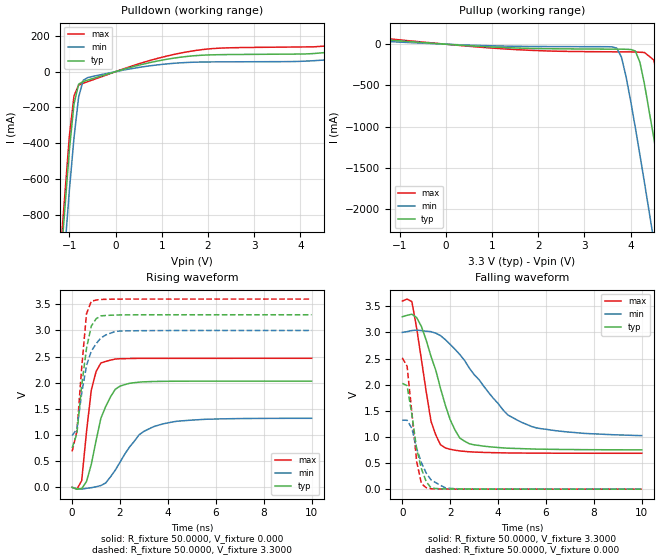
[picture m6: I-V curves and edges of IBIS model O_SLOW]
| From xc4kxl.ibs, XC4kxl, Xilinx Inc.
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|   Model O_SLOW
[Model]   O_SLOW
Model_type   Output
Polarity   Non-Inverting
Vmeas =   1.6500V
Cref =  50.0000pF
Rref =   1.0000M
Vref =  0.000V
C_comp   7.0000pF   6.0000pF   8.0000pF
[Temperature Range]   27.0000   100.0000   0.000
[Voltage Range]   3.3000V   3.0000V   3.6000V
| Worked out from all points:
|   slope of the pulldown table from 0 to 0.495 V, typ, clamps not added: 13.9 ohm
|   slope of the pullup table from 0 to 0.495 V, typ, clamps not added: 27.1 ohm
|   rising waveform, R_fixture 50.0000, V_fixture 0.000: 20-80 % time 708ps typ, 1.25ns min, 387ps max; typ from 0 V to 2.03 V
|   rising waveform, R_fixture 50.0000, V_fixture 3.3000: 20-80 % time 413ps typ, 515ps min, 309ps max; typ from 0.751 V to 3.3 V
|   falling waveform, R_fixture 50.0000, V_fixture 3.3000: 20-80 % time 1.03ns typ, 2.06ns min, 600ps max; typ from 3.3 V to 0.752 V
|   falling waveform, R_fixture 50.0000, V_fixture 0.000: 20-80 % time 461ps typ, 610ps min, 335ps max; typ from 2.02 V to 0 V
[Pulldown]
| voltage   I(typ)   I(min)   I(max)
-3.3V     -8.627A    -8.838A    -8.552A
-1.5V     -2.118A    -2.351A    -2.033A
-1V       -436.6mA   -662mA     -358.9mA
-900mV    -180.8mA   -369.1mA   -134.7mA
-800mV    -70.38mA   -141.6mA   -75.77mA
-700mV    -54.92mA   -48.08mA   -64.92mA
-600mV    -46.83mA   -33mA      -55.57mA
600mV     42.12mA    27.32mA    51.67mA
1.6V      86.5mA     51.89mA    113mA
2.3V      95.03mA    54.68mA    131.9mA
4.5V      106mA      64.68mA    142.4mA
6.6V      185.5mA    118.2mA    239.9mA
[Pullup]
| voltage   I(typ)   I(min)   I(max)
-3.3V     139.4mA    93.05mA    175.1mA
3.7V      -59.9mA    -48.13mA   -92.59mA
3.8V      -60.3mA    -155.1mA   -92.88mA
3.9V      -61.55mA   -391.7mA   -93.16mA
4.1V      -81.44mA   -1.009A    -94.6mA
4.2V      -218.1mA   -1.343A    -97.2mA
4.3V      -487mA     -1.684A    -101mA
4.5V      -1.135A    -2.381A    -191.2mA
4.7V      -1.825A    -3.088A    -749.8mA
4.9V      -2.532A    -3.801A    -1.425A
5.1V      -3.246A    -4.519A    -2.126A
6.6V      -8.69A     -9.964A    -7.553A
[Ramp]
| variable   typ   min   max
dV/dt_r   1.1778/0.6374n   0.7470/1.2967n   1.4802/0.3854n
dV/dt_f   1.5286/0.9702n   1.1850/2.1524n   1.7479/0.5879n
R_load = 50.0000
[Rising Waveform]
R_fixture = 50.0000
V_fixture = 0.000
| time   V(typ)   V(min)   V(max)
0s        0V         0V         0V
200ps     -34.28mV   -25.59mV   -34.33mV
400ps     -24.33mV   -34.12mV   129.9mV
600ps     111.5mV    -18.21mV   1.058V
800ps     439mV      -6.026mV   1.859V
1.2ns     1.32V      35.15mV    2.377V
1.8ns     1.874V     328.4mV    2.453V
2.8ns     2.012V     1.007V     2.465V
3.4ns     2.023V     1.16V      2.466V
10ns      2.03V      1.32V      2.467V
[Rising Waveform]
R_fixture = 50.0000
V_fixture = 3.3000
V_fixture_min = 3.0000
V_fixture_max = 3.6000
| time   V(typ)   V(min)   V(max)
0s        750.6mV    990.1mV    686.6mV
200ps     1.03V      1.117V     1.071V
400ps     1.945V     1.795V     2.29V
600ps     2.655V     2.327V     3.318V
800ps     3.082V     2.603V     3.556V
1ns       3.221V     2.744V     3.58V
1.2ns     3.278V     2.856V     3.592V
1.6ns     3.289V     2.946V     3.596V
2ns       3.296V     2.989V     3.598V
10ns      3.299V     2.999V     3.599V
[Falling Waveform]
R_fixture = 50.0000
V_fixture = 3.3000
V_fixture_min = 3.0000
V_fixture_max = 3.6000
| time   V(typ)   V(min)   V(max)
0s        3.3V       3V         3.6V
400ps     3.349V     3.035V     3.588V
800ps     3.11V      3.034V     2.474V
1.2ns     2.538V     3.014V     1.296V
1.8ns     1.603V     2.86V      789mV
2.2ns     1.133V     2.678V     746.1mV
2.6ns     918.3mV    2.463V     723.4mV
4.4ns     784.1mV    1.422V     693.3mV
5ns       775.2mV    1.276V     691.2mV
10ns      752.3mV    1.025V     686.9mV
[Falling Waveform]
R_fixture = 50.0000
V_fixture = 0.000
| time   V(typ)   V(min)   V(max)
0s        2.025V     1.32V      2.513V
200ps     1.98V      1.319V     2.352V
400ps     1.428V     1.163V     1.46V
600ps     766.4mV    776.4mV    527.9mV
800ps     389.2mV    503.9mV    104.6mV
1ns       142.7mV    307mV      27.72mV
1.2ns     23.92mV    176.7mV    7.611mV
1.8ns     5.596mV    26.32mV    2.983mV
2ns       4.084mV    14.64mV    2.244mV
10ns      225.2uV    532.6uV    159.7uV
